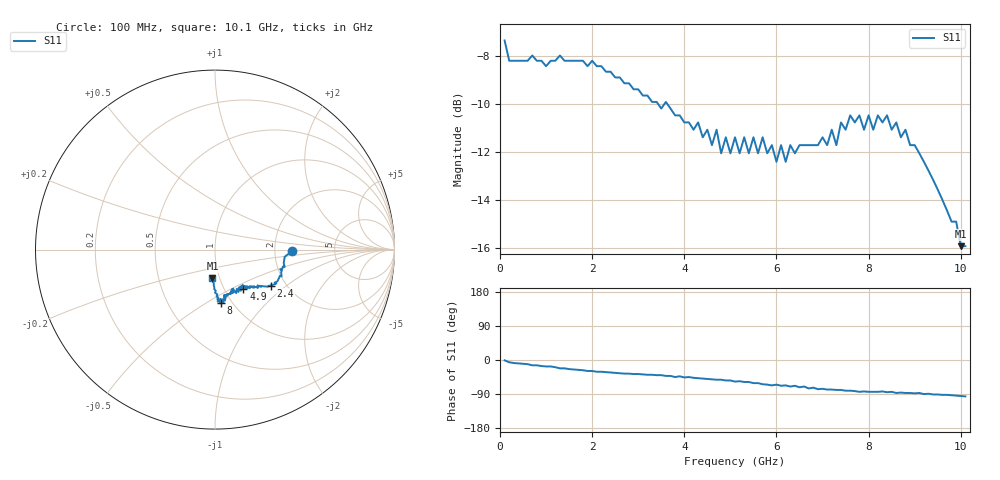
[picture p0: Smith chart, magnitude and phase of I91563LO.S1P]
!	IAM-91563 LO Port S PARAMETERS
!	Vd = 3 V LAST UPDATED 3-12-96
# ghz	s ma r	50
! Freq	LO(Mag)	LO(Ang)
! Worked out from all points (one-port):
!   101 points, 100 MHz to 10.1 GHz, reference 50 ohm
!   lowest |S11| = -15.9 dB at 10 GHz (marker M1), VSWR 1.38, Z = 46.2 - j15.1 ohm
!   |S11| at or under -10 dB: 3.437 GHz to 3.563 GHz (125.3 MHz wide, 3.58 % of centre); 3.637 GHz to end of sweep
!   S11 on the Smith chart (normalised r, x): 100 MHz: 2.51, -0.05; 2.4 GHz: 1.67, -0.78; 4.9 GHz: 1.23, -0.58; 8 GHz: 0.89, -0.58; 10.1 GHz: 0.92, -0.30
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0.1  0.43 -1.0
0.2  0.39 -6.0
1.4  0.39 -22.0
2.4  0.37 -33.0
2.6  0.36 -35.0
3.9  0.3 -43.0
4.6  0.26 -51.0
4.7  0.28 -52.0
4.8  0.25 -52.0
4.9  0.27 -54.0
5  0.25 -54.0
5.1  0.27 -57.0
5.2  0.25 -56.0
5.3  0.27 -58.0
5.4  0.25 -58.0
5.5  0.27 -61.0
6  0.24 -65.0
6.1  0.26 -68.0
6.4  0.25 -68.0
7.2  0.28 -78.0
7.3  0.26 -79.0
7.6  0.3 -81.0
7.9  0.28 -83.0
8  0.3 -84.0
8.9  0.26 -87.0
9.9  0.18 -94.0
10  0.16 -95.0
10.1  0.16 -96.0
